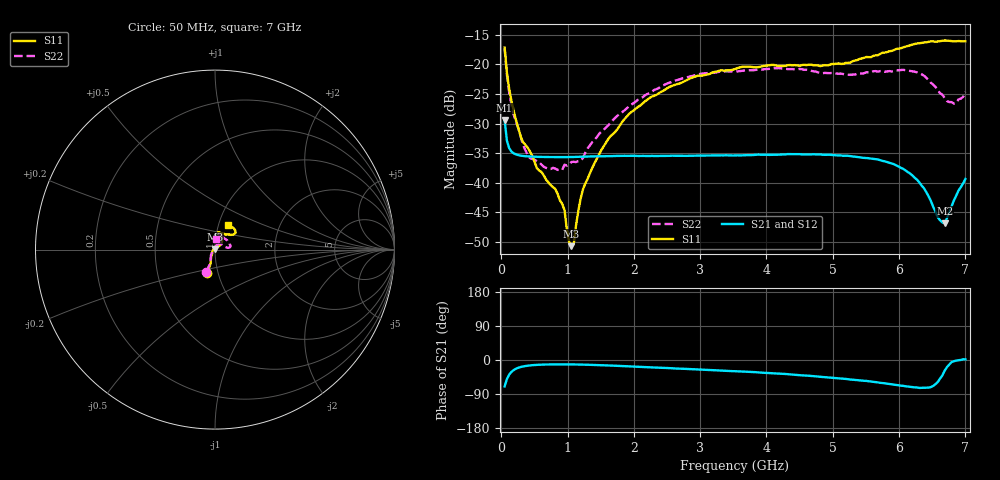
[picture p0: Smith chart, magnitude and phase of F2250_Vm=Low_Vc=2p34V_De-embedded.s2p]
! Integrated Device Technology
! Corporate Headquarters
! 6024 Silver Creek Valley Road
! San Jose, CA 95138  USA
! Phone:  1-408-284-8200
! Toll Free:  1-800-223-1366
! Webpage:  http://www.idt.com/
! Timing and RF Division
! 515 Groton Road, Suite 102
! Westford, MA 01886-6024
! Device:  F2250
! Description: Voltage Variable RF Attenuator
! Frequency:  50.0 -  6000.00 MHz
! Package:  3x3 mm Thin QFN Plastic Package: 16 pin
! Ports:  2 RF, 3 DC
!  Pin  1  = GND
!  Pin  2  = NC
!  Pin  3  = RF1  = Port 1
!  Pin  4  = NC
!  Pin  5  = GND
!  Pin  6  = GND
!  Pin  7  = GND
!  Pin  8  = GND
!  Pin  9  = NC
!  Pin 10  = RF2  = Port 2
!  Pin 11  = NC
!  Pin 12  = GND
!  Pin 13  = GND
!  Pin 14  = VCNTRL
!  Pin 15  = VDD
!  Pin 16  = VMODE
! Vcntrl:  2.340 Volts
! Vmode:  +0.000 Volts
! Vdd:  +3.30  Volts
! Current:  1.177 mA
! Data:  The device was measured on a the F2250 evaluation board which has
!  individual transmission lines to the RF pins.  Data was collected
!  using a calibrated network analyzer.  The evaluation board was
!  de-embedded using a TRL calibration technique.
!  The reference plane is the edge of the package pin.
! Misc:  SN 10
!  Action Tracker AT0258
! Date Measured:  2014-11-26
! Date:  2015-10-15  MJV
! Note:
!  Integrated Device Technology supplies this data as a sample of measured
!  data at the package pin for this product.  Your particular data for this
!  product may vary.
!  Data was taken at 25 degrees C.
!  Integrated Device Technology reserves the right to change this data at anytime.
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# GHz S dB R 50
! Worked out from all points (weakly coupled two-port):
!   201 points, 50 MHz to 7 GHz, reference 50 ohm
!   highest |S21| = -29.41 dB at 50 MHz (marker M1); lowest = -46.8 dB at 6.687 GHz (marker M2)
!   lowest |S11| = -50.7 dB at 1.058 GHz (marker M3), VSWR 1.01, Z = 49.8 + j0.241 ohm
!   |S11| at or under -10 dB: start of sweep to end of sweep
!   |S22| runs from -37.8 to -17.3 dB; largest |S21 - S12| = 6.8e-05
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0.05  -17.18 -108.6  -29.41 -69.7  -29.41 -69.7  -17.30 -110.9
0.08475  -21.45 -107.5  -32.91 -50.3  -32.91 -50.3  -21.79 -109.9
0.15425  -26.23 -116.5  -34.74 -31.1  -34.74 -31.1  -26.88 -121.9
0.29325  -32.21 -127.8  -35.41 -18.5  -35.41 -18.4  -32.25 -136.7
0.3975  -34.07 -141.8  -35.54 -15.0  -35.54 -15.0  -35.30 -159.8
0.91875  -43.55 158.0  -35.67 -11.5  -35.67 -11.5  -37.83 132.2
0.9535  -44.62 170.1  -35.67 -11.5  -35.66 -11.5  -36.94 129.8
1.023  -49.96 144.3  -35.66 -11.6  -35.65 -11.6  -36.84 114.4
1.05775  -50.69 124.3  -35.65 -11.6  -35.65 -11.6  -36.49 109.1
1.0925  -50.37 88.8  -35.64 -11.7  -35.64 -11.7  -36.45 104.5
1.162  -44.71 56.6  -35.62 -11.9  -35.62 -11.9  -36.34 93.6
1.2315  -41.12 44.6  -35.59 -12.1  -35.59 -12.1  -35.85 84.1
1.61375  -32.61 40.9  -35.51 -14.5  -35.51 -14.5  -30.30 64.6
1.9265  -28.40 41.3  -35.45 -16.9  -35.45 -16.9  -27.09 56.1
2.37825  -24.88 47.3  -35.46 -20.3  -35.46 -20.3  -24.00 56.4
3.525  -20.80 72.5  -35.39 -29.6  -35.39 -29.6  -21.23 74.5
4.7065  -20.17 72.3  -35.19 -42.6  -35.19 -42.6  -21.19 72.1
5.85325  -17.82 40.5  -36.62 -63.3  -36.62 -63.3  -21.16 22.7
6.27025  -16.50 40.1  -39.47 -72.6  -39.49 -72.7  -21.37 9.4
6.68725  -15.99 48.8  -46.83 -28.2  -46.78 -27.6  -25.69 28.2
6.861  -16.13 55.1  -42.18 -1.5  -42.13 -1.5  -26.54 57.9
7  -16.12 63.2  -39.35 1.7  -39.30 1.6  -24.67 83.2
